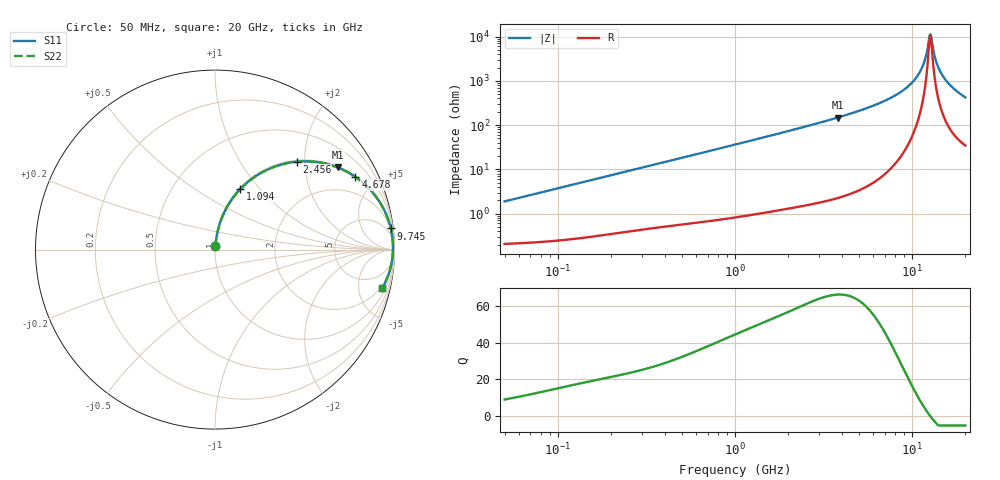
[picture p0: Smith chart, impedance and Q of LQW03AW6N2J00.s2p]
!Murata Part Number: LQW03AW6N2J00
!These Parameters are Measured in Series Mode Connection
!  o--[Z]--o
!Port1  Port2
!  o-------o
!Freq. Start=50[MHz] Stop=20[GHz], 401[Steps]
# Hz S RI R 50
!Freq.(Hz) S11(Real) S11(Imag) S21(Real) S21(Imag) S12(Real) S12(Imag) S22(Real) S22(Imag)
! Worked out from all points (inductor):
!   401 points, 50 MHz to 20 GHz, reference 50 ohm
!   read as one part in series: L = 5.97 nH near 51.52 MHz
!   highest Q = 66 at 3.793 GHz (marker M1), where L = 6.21 nH
!   self-resonance near 12.57 GHz
!   S11 on the Smith chart (normalised r, x): 50 MHz: 1.00, +0.04; 1.094 GHz: 1.02, +0.79; 2.456 GHz: 1.03, +1.82; 4.678 GHz: 1.06, +3.83; 9.745 GHz: 2, +16; 20 GHz: 1.69, -8.43
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5e7  0.00242 0.0187  0.9976 -0.0187  0.9976 -0.0187  0.00242 0.0187
1.364002e8  0.00536 0.0503  0.9946 -0.0503  0.9946 -0.0503  0.00536 0.0503
3.721004e8  0.0228 0.1323  0.9772 -0.1323  0.9772 -0.1323  0.0228 0.1323
1e9  0.1217 0.3158  0.8783 -0.3158  0.8783 -0.3158  0.1217 0.3158
1.094034e9  0.1414 0.3377  0.8586 -0.3377  0.8586 -0.3377  0.1414 0.3377
1.614971e9  0.2612 0.4299  0.7388 -0.4299  0.7388 -0.4299  0.2612 0.4299
2.456456e9  0.4541 0.4897  0.5459 -0.4897  0.5459 -0.4897  0.4541 0.4897
2.728004e9  0.5095 0.492  0.4905 -0.492  0.4905 -0.492  0.5095 0.492
3.792786e9  0.6837 0.4575  0.3163 -0.4575  0.3163 -0.4575  0.6837 0.4575
4.677679e9  0.7825 0.4048  0.2175 -0.4048  0.2175 -0.4048  0.7825 0.4048
7.442007e9  0.9356 0.2336  0.0644 -0.2336  0.0644 -0.2336  0.9356 0.2336
9.745021e9  0.9793 0.1179  0.0207 -0.1179  0.0207 -0.1179  0.9793 0.1179
1.066139e10  0.9869 0.0781  0.0131 -0.0781  0.0131 -0.0781  0.9869 0.0781
1.131968e10  0.99 0.0513  0.00997 -0.0513  0.00997 -0.0513  0.99 0.0513
1.183995e10  0.9914 0.0311  0.00864 -0.0311  0.00864 -0.0311  0.9914 0.0311
1.238412e10  0.9918 0.0107  0.00818 -0.0107  0.00818 -0.0107  0.9918 0.0107
1.276073e10  0.9916 -0.00292  0.00838 0.00292  0.00838 0.00292  0.9916 -0.00292
1.295331e10  0.9914 -0.00977  0.00864 0.00977  0.00864 0.00977  0.9914 -0.00977
1.375312e10  0.9893 -0.0373  0.0107 0.0373  0.0107 0.0373  0.9893 -0.0373
1.482269e10  0.9843 -0.072  0.0157 0.072  0.0157 0.072  0.9843 -0.072
1.696185e10  0.9677 -0.1357  0.0323 0.1357  0.0323 0.1357  0.9677 -0.1357
2e10  0.9313 -0.2152  0.0687 0.2152  0.0687 0.2152  0.9313 -0.2152
